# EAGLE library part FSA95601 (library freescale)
Digital Audio Amplifier Controller Source: http://www.freescale.com/files/dsp/doc/prod_brief/FSA95601PB.pdf
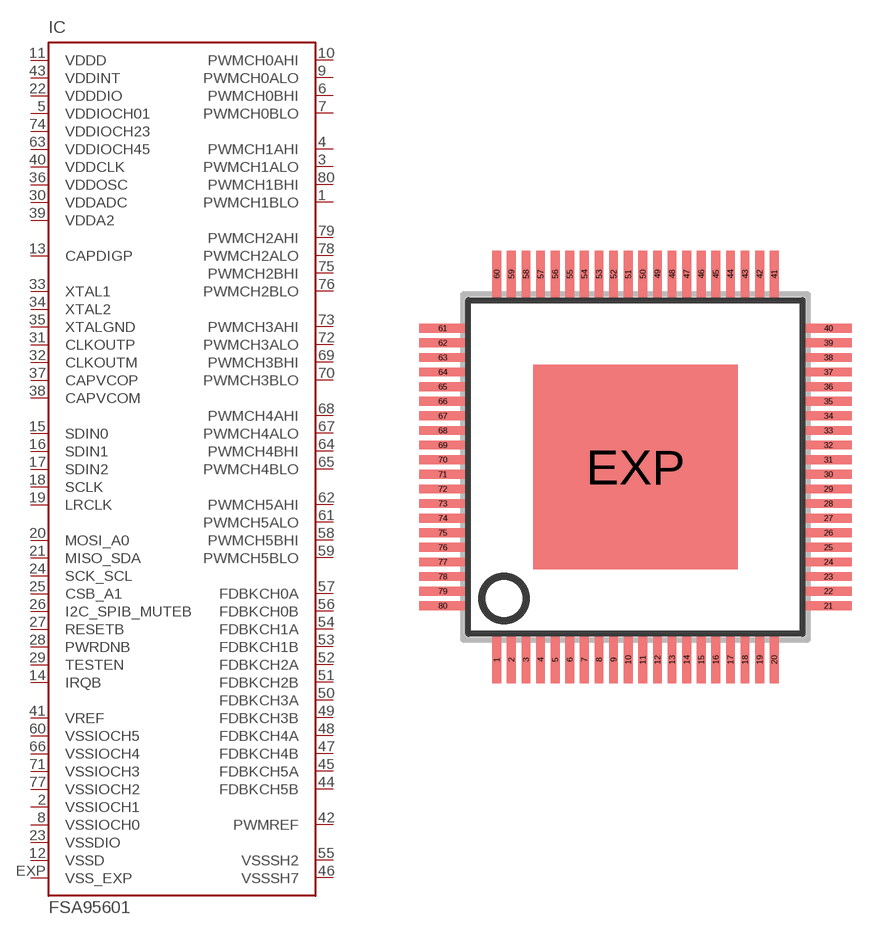
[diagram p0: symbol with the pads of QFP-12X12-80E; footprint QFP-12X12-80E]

Designator prefix IC

## FSA95601 (MPN: FSA95601AH; OC_FARNELL: unknown; OC_NEWARK: 69M3598)  [QFP-12X12-80E]
1  PWMCH1BLO  out
2  VSSIOCH1  in
3  PWMCH1ALO  out
4  PWMCH1AHI  out
5  VDDIOCH01  in
6  PWMCH0BHI  out
7  PWMCH0BLO  out
8  VSSIOCH0  in
9  PWMCH0ALO  out
10  PWMCH0AHI  out
11  VDDD  in
12  VSSD  in
13  CAPDIGP  out
14  IRQB  out
15  SDIN0  in
16  SDIN1  in
17  SDIN2
18  SCLK  in
19  LRCLK  in
20  MOSI_A0  in
21  MISO_SDA
22  VDDDIO  in
23  VSSDIO  in
24  SCK_SCL  in
25  CSB_A1  in
26  I2C_SPIB_MUTEB  in
27  RESETB  in
28  PWRDNB  in
29  TESTEN  in
30  VDDADC  in
31  CLKOUTP  out
32  CLKOUTM  out
33  XTAL1  in
34  XTAL2  in
35  XTALGND  in
36  VDDOSC  in
37  CAPVCOP  out
38  CAPVCOM  in
39  VDDA2  in
40  VDDCLK  in
41  VREF  out
42  PWMREF  in
43  VDDINT  in
44  FDBKCH5B  in
45  FDBKCH5A  in
46  VSSSH7  in
47  FDBKCH4B  in
48  FDBKCH4A  in
49  FDBKCH3B  in
50  FDBKCH3A  in
51  FDBKCH2B  in
52  FDBKCH2A  in
53  FDBKCH1B  in
54  FDBKCH1A  in
55  VSSSH2  in
56  FDBKCH0B  in
57  FDBKCH0A  in
58  PWMCH5BHI  out
59  PWMCH5BLO  out
60  VSSIOCH5  in
61  PWMCH5ALO  out
62  PWMCH5AHI  out
63  VDDIOCH45  in
64  PWMCH4BHI  out
65  PWMCH4BLO  out
66  VSSIOCH4  in
67  PWMCH4ALO  out
68  PWMCH4AHI  out
69  PWMCH3BHI  out
70  PWMCH3BLO  out
71  VSSIOCH3  in
72  PWMCH3ALO  out
73  PWMCH3AHI  out
74  VDDIOCH23  in
75  PWMCH2BHI  out
76  PWMCH2BLO  out
77  VSSIOCH2  in
78  PWMCH2ALO  out
79  PWMCH2AHI  out
80  PWMCH1BHI  out
EXP  VSS_EXP  in

## Footprint QFP-12X12-80E (pad centres in mm)
QFP80 quad flat pack, square
smd 0.3 x 1.6: 1 -4.75,-6.6; 2 -4.25,-6.6; 3 -3.75,-6.6; 4 -3.25,-6.6; 5 -2.75,-6.6; 6 -2.25,-6.6; 7 -1.75,-6.6; 8 -1.25,-6.6; 9 -0.75,-6.6; 10 -0.25,-6.6; 11 0.25,-6.6; 12 0.75,-6.6; 13 1.25,-6.6; 14 1.75,-6.6; 15 2.25,-6.6; 16 2.75,-6.6; 17 3.25,-6.6; 18 3.75,-6.6; 19 4.25,-6.6; 20 4.75,-6.6; 41 4.75,6.6; 42 4.25,6.6; 43 3.75,6.6; 44 3.25,6.6; 45 2.75,6.6; 46 2.25,6.6; 47 1.75,6.6; 48 1.25,6.6; 49 0.75,6.6; 50 0.25,6.6; 51 -0.25,6.6; 52 -0.75,6.6; 53 -1.25,6.6; 54 -1.75,6.6; 55 -2.25,6.6; 56 -2.75,6.6; 57 -3.25,6.6; 58 -3.75,6.6; 59 -4.25,6.6; 60 -4.75,6.6
smd 1.6 x 0.3: 21 6.6,-4.75; 22 6.6,-4.25; 23 6.6,-3.75; 24 6.6,-3.25; 25 6.6,-2.75; 26 6.6,-2.25; 27 6.6,-1.75; 28 6.6,-1.25; 29 6.6,-0.75; 30 6.6,-0.25; 31 6.6,0.25; 32 6.6,0.75; 33 6.6,1.25; 34 6.6,1.75; 35 6.6,2.25; 36 6.6,2.75; 37 6.6,3.25; 38 6.6,3.75; 39 6.6,4.25; 40 6.6,4.75; 61 -6.6,4.75; 62 -6.6,4.25; 63 -6.6,3.75; 64 -6.6,3.25; 65 -6.6,2.75; 66 -6.6,2.25; 67 -6.6,1.75; 68 -6.6,1.25; 69 -6.6,0.75; 70 -6.6,0.25; 71 -6.6,-0.25; 72 -6.6,-0.75; 73 -6.6,-1.25; 74 -6.6,-1.75; 75 -6.6,-2.25; 76 -6.6,-2.75; 77 -6.6,-3.25; 78 -6.6,-3.75; 79 -6.6,-4.25; 80 -6.6,-4.75
smd 7 x 7: EXP 0,0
